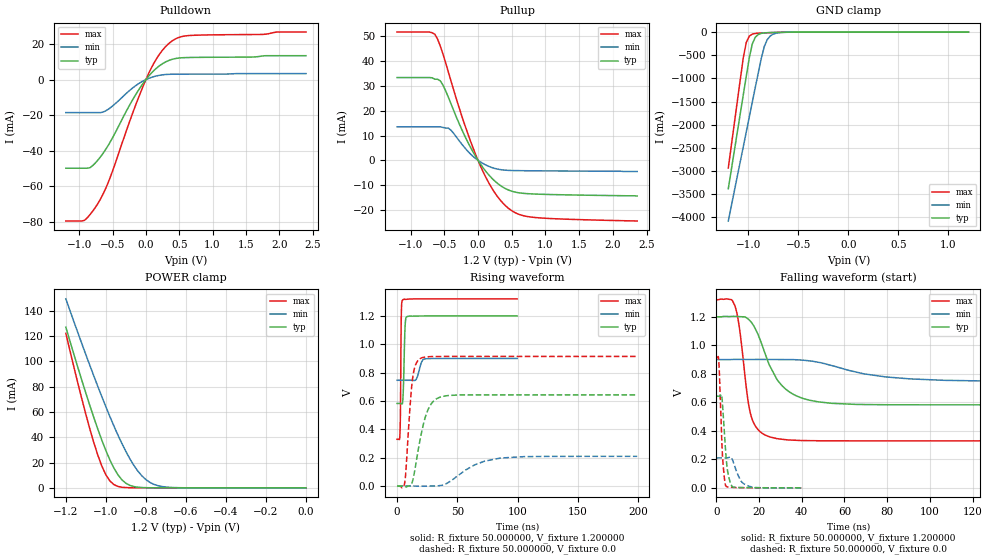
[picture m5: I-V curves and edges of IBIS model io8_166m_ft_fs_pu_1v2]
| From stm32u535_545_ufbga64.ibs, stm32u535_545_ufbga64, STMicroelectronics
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|   Model io8_166m_ft_fs_pu_1v2
[Model]  io8_166m_ft_fs_pu_1v2
Model_type I/O
Polarity   Non-Inverting
Enable   Active-Low
Vinl =   0.360000V
Vinh =   0.840000V
Vmeas =  0.600000V
Cref =   50.000000pF
Rref =   100.000000M
Vref =   0.0V
C_comp   3.151500pF   3.086800pF   3.197700pF
[Temperature Range]   25.000000   0.140000k   -40.000000
[Pullup Reference]   1.200000V   0.900000V   1.320000V
[Pulldown Reference]   0.0V   0.0V   0.0V
[POWER Clamp Reference]   1.200000V   0.900000V   1.320000V
[GND Clamp Reference]   0.0V   0.0V   0.0V
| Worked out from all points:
|   slope of the pulldown table from 0 to 0.18 V, typ, clamps not added: 25.4 ohm
|   slope of the pullup table from 0 to 0.18 V, typ, clamps not added: 27.8 ohm
|   GND clamp passes 1 mA (typ) near -0.51 V on its own axis
|   POWER clamp passes 1 mA (typ) near -0.86 V on its own axis
|   rising waveform, R_fixture 50.000000, V_fixture 1.200000: 20-80 % time 1.12ns typ, 3.01ns min, 569ps max; typ from 0.583 V to 1.2 V
|   rising waveform, R_fixture 50.000000, V_fixture 0.0: 20-80 % time 9.51ns typ, 24.6ns min, 4.59ns max; typ from 0 V to 0.643 V
|   falling waveform, R_fixture 50.000000, V_fixture 1.200000: 20-80 % time 12ns typ, 29.3ns min, 5.07ns max; typ from 1.2 V to 0.583 V
|   falling waveform, R_fixture 50.000000, V_fixture 0.0: 20-80 % time 1.95ns typ, 3.63ns min, 1.47ns max; typ from 0.643 V to 0 V
[Pulldown]
|Voltage   I(typ)   I(min)   I(max)
-1.2V     -49.86mA   -18.57mA   -79.56mA
-920mV    -49.86mA   -18.57mA   -79.19mA
-840mV    -49.6mA    -18.57mA   -76.08mA
-720mV    -45.32mA   -18.57mA   -69.74mA
-560mV    -36.71mA   -16.58mA   -57.44mA
-200mV    -11.43mA   -4.74mA    -19.03mA
0V        0A         0A         0A
160mV     6.477mA    2.075mA    11.78mA
360mV     10.99mA    2.99mA     20.81mA
480mV     12.07mA    3.054mA    23.52mA
640mV     12.43mA    3.075mA    24.76mA
2.4V      13.45mA    3.36mA     26.76mA
[Pullup]
|Voltage   I(typ)   I(min)   I(max)
-1.2V     33.39mA    13.53mA    51.75mA
-640mV    32.72mA    13.53mA    50.87mA
-560mV    32.1mA     13.53mA    46.17mA
-520mV    30.37mA    13.28mA    42.92mA
-400mV    22.74mA    12.14mA    31.92mA
-240mV    12.39mA    6.508mA    17.85mA
0V        580fA      234pA      0A
200mV     -7.072mA   -2.851mA   -11mA
440mV     -11.84mA   -4.03mA    -19.1mA
600mV     -13.07mA   -4.154mA   -21.71mA
840mV     -13.59mA   -4.223mA   -23.04mA
2.36V     -14.4mA    -4.5mA     -24.47mA
[GND_clamp]
|Voltage   I(typ)   I(min)   I(max)
-1.2V     -3.379A    -4.076A    -2.932A
-1.05V    -1.35A     -2.47A     -550.7mA
-1.02V    -947.8mA   -2.149A    -221.5mA
-990mV    -552.4mA   -1.829A    -88.44mA
-960mV    -255.3mA   -1.51A     -44.87mA
-930mV    -111.8mA   -1.191A    -30.68mA
-870mV    -28.36mA   -564.6mA   -21.34mA
-840mV    -18.65mA   -309.5mA   -18.49mA
-810mV    -14.07mA   -161.6mA   -15.92mA
-780mV    -11.37mA   -83.33mA   -13.53mA
-600mV    -3.009mA   -4.322mA   -3.091mA
1.2V      0A         13.65nA    0A
[POWER_clamp]
|Voltage   I(typ)   I(min)   I(max)
-1.2V     127mA      149.4mA    122.2mA
-1.12V    84.98mA    114mA      70.29mA
-1.06V    55.52mA    88.42mA    35.69mA
-1.02V    37.64mA    72.04mA    17.19mA
-1V       29.52mA    64.13mA    10.33mA
-960mV    15.7mA     48.99mA    2.596mA
-900mV    3.636mA    28.77mA    207.8uA
-840mV    502.9uA    13.24mA    43.45uA
-800mV    129uA      6.535mA    43.45uA
-740mV    26.2uA     1.726mA    43.45uA
-620mV    25.1uA     82.33uA    35.72uA
0V        0A         17.36nA    0A
[Ramp]
| variable   typ   min   max
dV/dt_r  0.38568/9.50395n   0.12561/24.60184n   0.54819/4.57784n
dV/dt_f  0.37043/11.97971n   92.35200m/29.34628n 0.59405/5.05410n
R_load = 50.000000
[Rising Waveform]
R_fixture= 50.000000
V_fixture= 1.200000
V_fixture_min= 0.900000
V_fixture_max= 1.320000
|time   V(typ)   V(min)   V(max)
0s        582.6mV    746mV      329.9mV
2.402ns   582.7mV    746mV      368.3mV
2.803ns   582.7mV    746mV      519.1mV
3.203ns   582.3mV    746mV      967.4mV
3.604ns   580.9mV    746mV      1.24V
4.605ns   589.8mV    746mV      1.312V
6.607ns   1.116V     746.1mV    1.316V
8.008ns   1.193V     746.1mV    1.317V
22.82ns   1.2V       896.8mV    1.32V
99.7ns    1.2V       900mV      1.32V
[Rising Waveform]
R_fixture= 50.000000
V_fixture= 0.0
V_fixture_min= 0.0
V_fixture_max= 0.0
|time   V(typ)   V(min)   V(max)
0s        435.6uV    496.7uV    380uV
6.406ns   -3.122mV   496uV      27.19mV
10.81ns   2.254mV    499uV      564.7mV
12.81ns   34.17mV    532.7uV    754mV
15.22ns   136.6mV    192uV      852.4mV
19.22ns   332.6mV    -655.5uV   898.9mV
26.83ns   558.3mV    589.6uV    912.5mV
37.64ns   631.9mV    6.715mV    913.9mV
86.09ns   643.2mV    197.9mV    914mV
199.4ns   643.3mV    210mV      914mV
[Falling Waveform]
R_fixture= 50.000000
V_fixture= 1.200000
V_fixture_min= 0.900000
V_fixture_max= 1.320000
|time   V(typ)   V(min)   V(max)
0s        1.2V       900mV      1.32V
8.809ns   1.203V     901.1mV    1.273V
10.81ns   1.201V     901.2mV    1.124V
16.02ns   1.168V     900.6mV    520.2mV
19.22ns   1.087V     900.8mV    414.2mV
25.23ns   850.4mV    900.5mV    356.8mV
35.64ns   659.7mV    899.6mV    335mV
54.05ns   593.2mV    857.9mV    330.1mV
90.49ns   582.7mV    764.7mV    329.9mV
199.4ns   582.6mV    746mV      329.9mV
[Falling Waveform]
R_fixture= 50.000000
V_fixture= 0.0
V_fixture_min= 0.0
V_fixture_max= 0.0
|time   V(typ)   V(min)   V(max)
0s        643.3mV    210mV      914mV
1.201ns   643.1mV    210mV      877.5mV
2.563ns   644.5mV    210mV      333.6mV
3.363ns   484.1mV    209.9mV    134.9mV
4.484ns   235.1mV    209.6mV    13.37mV
5.606ns   93.18mV    212.3mV    5.873mV
7.768ns   6.367mV    189.2mV    3.727mV
11.53ns   2.618mV    49.48mV    1.519mV
15.46ns   1.807mV    11.06mV    810.7uV
39.88ns   435.6uV    496.7uV    380uV
